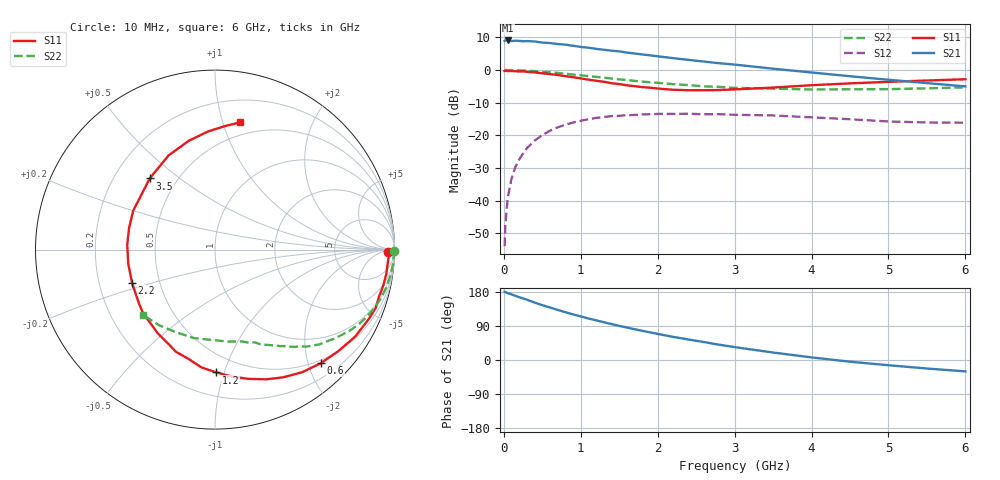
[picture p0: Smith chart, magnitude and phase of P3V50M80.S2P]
! SIEMENS Small Signal Semiconductors
! BFP181
! Si NPN RF Bipolar Junction Transistor in SOT143
! VCE = 0.5 V  IC = 0.8 mA
! Common Emitter S-Parameters:  March  1996
# GHz  S  MA  R  50
!  f  S11  S21  S12  S22
! GHz  MAG  ANG  MAG  ANG  MAG  ANG  MAG  ANG
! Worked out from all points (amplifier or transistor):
!   36 points, 10 MHz to 6 GHz, reference 50 ohm
!   highest |S21| = 9.1 dB at 50 MHz (marker M1)
!   |S21| within 3 dB of that: start of sweep to 1.352 GHz
!   unconditionally stable (mu >= 1): 2.878 GHz to end of sweep
!   at 250 MHz: K = 0.10, MSG = 17.2 dB, |S12| = -25.6 dB
!   at 1.4 GHz: K = 0.54, MSG = 10.0 dB, |S12| = -14.1 dB
!   at 6 GHz: K = 1.59, MAG = 1.1 dB, |S12| = -16.1 dB
!   S11 on the Smith chart (normalised r, x): 10 MHz: 48, -22; 600 MHz: 0.44, -2.22; 1.2 GHz: 0.37, -0.94; 2.2 GHz: 0.35, -0.17; 3.5 GHz: 0.35, +0.39; 6 GHz: 0.38, +1.14
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0.01  0.966 -0.9  2.798 179.7  0.002 81.2  0.9982 -0.4
0.02  0.9706 -1.6  2.836 179.3  0.0043 89.1  1 -0.9
0.05  0.966 -3.9  2.836 176.5  0.0109 88.6  0.9959 -2.2
0.1  0.964 -8.1  2.778 173.1  0.0216 84.7  0.9955 -4.2
0.15  0.9588 -12.2  2.814 169.3  0.0326 81.3  0.9916 -6.3
0.2  0.9506 -16.0  2.794 165.8  0.0426 79.0  0.9883 -8.5
0.3  0.9405 -24.2  2.774 159.2  0.0634 73.3  0.9772 -12.6
0.4  0.9193 -31.8  2.734 151.5  0.0827 68.0  0.9621 -16.7
0.6  0.8647 -47.1  2.587 138.6  0.1175 58.0  0.9234 -24.2
0.8  0.8066 -61.9  2.446 126.2  0.145 48.6  0.8768 -30.9
1.1  0.7118 -82.8  2.198 109.5  0.176 36.5  0.8058 -39.4
1.2  0.6843 -89.4  2.108 104.6  0.1846 32.4  0.7853 -42.3
1.5  0.6094 -111.0  1.929 90.0  0.1991 23.3  0.718 -48.6
1.7  0.5651 -124.4  1.79 81.3  0.205 17.8  0.6805 -52.6
1.9  0.536 -138.1  1.679 72.9  0.21 12.8  0.6488 -56.0
2.2  0.4978 -158.3  1.52 61.0  0.2125 6.6  0.6074 -61.0
2.8  0.4936 165.8  1.269 40.4  0.2103 -3.7  0.5523 -70.1
3.5  0.538 132.5  1.047 19.7  0.2011 -12.1  0.5177 -81.9
4  0.5851 116.2  0.916 6.9  0.1883 -16.9  0.5034 -92.2
4.5  0.6238 103.5  0.803 -4.5  0.1761 -21.0  0.5067 -103.5
5.5  0.6895 85.6  0.63 -22.5  0.157 -19.6  0.5239 -126.4
6  0.7223 78.9  0.561 -30.0  0.156 -18.1  0.5422 -137.9
